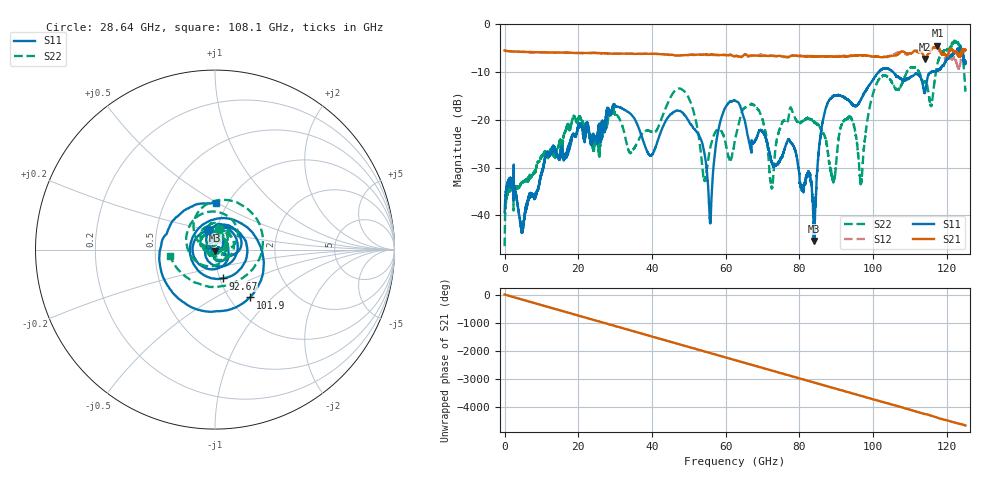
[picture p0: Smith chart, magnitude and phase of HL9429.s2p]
! 5/9/2023 1:24:54 PM
! H:\PROTOTYPE_DATA\110GHZ-ATTN\A2.S2P
! CHANNEL.1
! TR.MEASUREMENT
! CORRECTED.DATA
! RF.CORRECTION: FULL.TWO.PORT.CAL.PORT.1.2
! AVERAGING: 1 PointByPoint
! IF.BANDWIDTH: 1KHZ
! SWEEPTYPE:  FREQ.SWEEP(Linear)
! Reference Plane Port Info
! PORT:  PORT1  PORT2
! DISTANCE:  0  m  0  m
! TIME:  0  s  0  s
! PHASE.OFFSET:  0 °  0 °
! LOSS:  0  dB  0  dB
! REF.LOSS:  0  dB  0  dB
! REF.FREQ:  0  Hz  0  Hz
! Power Info
! POWER:  -10  dBm  -10  dBm
! EFF.POWER:  -10  dBm  -10  dBm
! POWER(>54G):  -10  dBm  -10  dBm
! EFF.POWER(>54G):  -10  dBm  -10  dBm
! SOURCE.ATTEN:  0  dB  0  dB
! TEST.ATTEN:  0  dB  0  dB
# GHZ S RI R 50.0
! FREQ.GHZ  S11RE  S11IM  S21RE  S21IM  S12RE  S12IM  S22RE  S22IM
!; PortSelection: Port_12
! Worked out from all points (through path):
!   10000 points, 12.5 MHz to 125 GHz, reference 50 ohm
!   highest |S21| = -4.46 dB at 117.4 GHz (marker M1); lowest = -7.2 dB at 114.1 GHz (marker M2)
!   group delay of S21, straight-line fit = 104 ps
!   lowest |S11| = -45.4 dB at 84 GHz (marker M3), VSWR 1.01, Z = 49.9 - j0.526 ohm
!   |S11| at or under -10 dB: start of sweep to 101.5 GHz; 105.4 GHz to 115.7 GHz (10.27 GHz wide, 9.29 % of centre); 115.7099 GHz to 115.7151 GHz (5.285 MHz wide, 0.00457 % of centre)
!   |S22| runs from -46.5 to -3.4 dB; largest |S21 - S12| = 0.17
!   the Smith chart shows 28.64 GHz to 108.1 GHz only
!   S11 on the Smith chart (normalised r, x): 28.64 GHz: 0.90, +0.20; 92.67 GHz: 1.03, -0.34; 101.9 GHz: 1.24, -0.74; 108.1 GHz: 0.89, +0.49
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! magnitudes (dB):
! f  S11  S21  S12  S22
! 12.5 MHz  -39.4  -5.5  -5.5  -46.5
! 20.85 GHz  -20.9  -6.0  -6.0  -20.0
! 28.64 GHz  -18.8  -6.1  -6.1  -18.9
! 41.67 GHz  -24.1  -6.2  -6.2  -21.5
! 48.76 GHz  -18.9  -6.4  -6.4  -14.0
! 55.76 GHz  -41.3  -6.4  -6.4  -25.9
! 62.51 GHz  -16.0  -6.7  -6.5  -24.2
! 68.24 GHz  -24.0  -6.5  -6.6  -17.3
! 72.44 GHz  -28.9  -6.6  -6.6  -34.1
! 75.41 GHz  -27.6  -6.7  -6.8  -20.4
! 83.34 GHz  -34.2  -6.7  -6.6  -20.0
! 84 GHz  -45.4  -6.7  -6.6  -20.4
! 87.1 GHz  -17.7  -6.7  -6.8  -24.2
! 89.21 GHz  -15.0  -6.8  -6.7  -32.9
! 92.67 GHz  -15.6  -6.7  -6.6  -19.8
! 96.69 GHz  -15.7  -6.5  -6.4  -33.3
! 101.9 GHz  -9.6  -6.9  -6.9  -11.1
! 104.2 GHz  -9.3  -6.7  -6.8  -11.2
! 108.1 GHz  -11.7  -5.7  -6.1  -11.8
! 114.1 GHz  -14.2  -7.2  -7.3  -12.0
! 117.4 GHz  -9.5  -4.5  -4.9  -8.2
! 125 GHz  -8.2  -5.4  -5.2  -14.1
